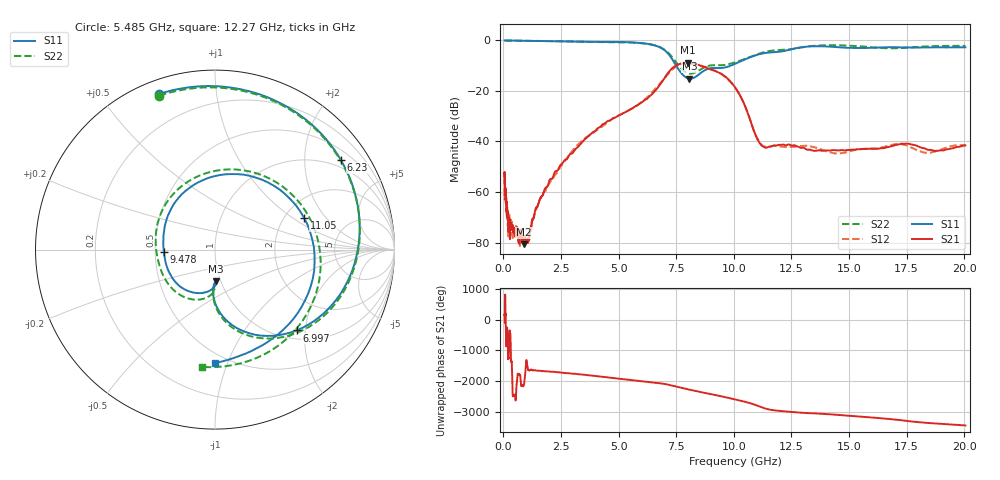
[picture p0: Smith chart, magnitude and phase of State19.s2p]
# Hz S DB R 50
!freq MagS11 AngS11 MagS21 AngS21 MagS12 AngS12 MagS22 AngS22
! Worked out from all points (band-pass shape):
!   1601 points, 50 MHz to 20.05 GHz, reference 50 ohm
!   highest |S21| = -8.83 dB at 8.008 GHz (marker M1); lowest = -80.6 dB at 881.5 MHz (marker M2)
!   |S21| within 3 dB of the highest: 7.24 GHz to 9.102 GHz (1.863 GHz wide, 22.8 % of centre)
!   lowest |S11| = -15.1 dB at 8.068 GHz (marker M3), VSWR 1.43, Z = 47.4 - j17.2 ohm
!   |S11| at or under -10 dB: 7.499 GHz to 9.858 GHz (2.359 GHz wide, 27.2 % of centre)
!   |S22| runs from -13.1 to 0.0 dB; largest |S21 - S12| = 0.022
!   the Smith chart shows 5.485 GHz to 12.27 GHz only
!   S11 on the Smith chart (normalised r, x): 5.485 GHz: 0.06, +0.70; 6.23 GHz: 0.76, +2.94; 6.997 GHz: 1.18, -1.80; 9.478 GHz: 0.56, -0.02; 11.05 GHz: 2.55, +1.24; 12.27 GHz: 0.43, -0.90
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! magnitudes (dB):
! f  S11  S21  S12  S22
! 50 MHz  0.0  -52.5  -54.6  0.0
! 52.3 MHz  0.0  -54.3  -62.1  0.0
! 82.91 MHz  0.0  -59.1  -59.0  0.0
! 135.9 MHz  0.0  -66.9  -67.6  0.0
! 206 MHz  0.0  -69.5  -75.2  0.0
! 250.4 MHz  0.0  -71.6  -69.2  0.0
! 281.2 MHz  0.0  -78.7  -72.3  0.0
! 369.6 MHz  0.0  -74.1  -73.1  0.0
! 881.5 MHz  -0.1  -80.6  -77.2  -0.1
! 1.005 GHz  -0.1  -80.0  -79.6  -0.1
! 2.722 GHz  -0.3  -47.2  -46.9  -0.4
! 5.485 GHz  -0.7  -27.3  -27.4  -0.8
! 6.23 GHz  -1.3  -23.1  -22.5  -1.4
! 6.997 GHz  -3.9  -14.8  -14.9  -3.7
! 7.402 GHz  -8.5  -10.4  -11.0  -7.5
! 8.008 GHz  -15.0  -8.8  -9.1  -13.0
! 8.068 GHz  -15.1  -8.9  -9.1  -13.1
! 9.478 GHz  -10.9  -13.3  -13.4  -9.8
! 10.22 GHz  -8.6  -20.9  -20.9  -8.1
! 11.05 GHz  -5.6  -39.6  -39.4  -5.3
! 12.27 GHz  -4.0  -41.5  -42.2  -3.6
! 20.05 GHz  -2.7  -41.6  -41.4  -2.1
